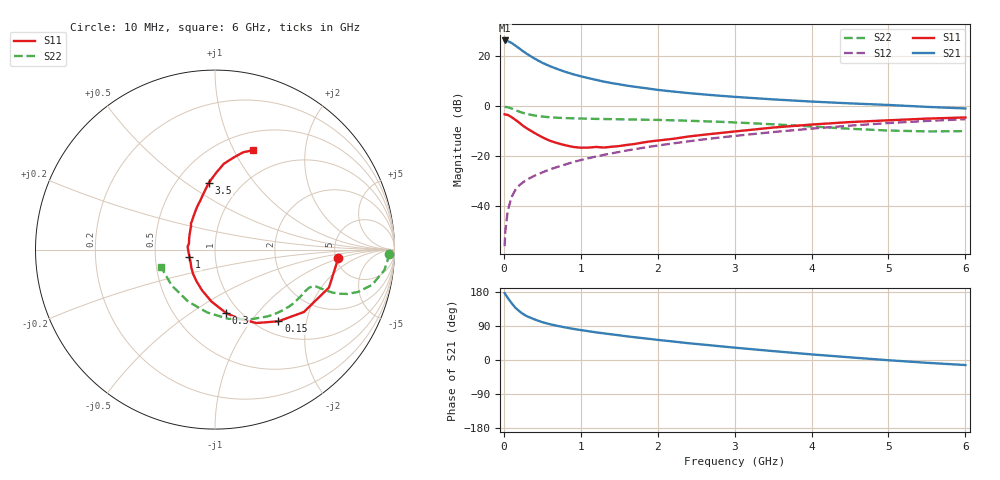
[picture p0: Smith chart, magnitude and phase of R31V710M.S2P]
! SIEMENS Small Signal Semiconductors
! BFR181
! Si NPN RF Bipolar Junction Transistor in SOT23
! VCE = 1.75 V  IC = 10 mA
! Common Emitter S-Parameters:  May  1996
# GHz  S  MA  R  50
!  f  S11  S21  S12  S22
! GHz  MAG  ANG  MAG  ANG  MAG  ANG  MAG  ANG
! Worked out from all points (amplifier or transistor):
!   36 points, 10 MHz to 6 GHz, reference 50 ohm
!   highest |S21| = 26.2 dB at 10 MHz (marker M1)
!   |S21| within 3 dB of that: start of sweep to 193.1 MHz
!   unconditionally stable (mu >= 1): 599.6 MHz to 2.801 GHz
!   at 250 MHz: K = 0.66, MSG = 26.2 dB, |S12| = -30.4 dB
!   at 1.4 GHz: K = 1.11, MAG = 12.0 dB, |S12| = -18.9 dB
!   at 6 GHz: K = 0.88, MSG = 2.1 dB, |S12| = -5.2 dB
!   S11 on the Smith chart (normalised r, x): 10 MHz: 5.23, -0.93; 150 MHz: 1.24, -1.38; 300 MHz: 0.87, -0.70; 1 GHz: 0.75, -0.06; 3.5 GHz: 0.71, +0.62; 6 GHz: 0.70, +1.20
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0.01  0.6877 -3.9  20.5 176.7  0.0016 92.2  0.9719 -1.3
0.02  0.6796 -7.6  20.31 173.3  0.0033 86.6  0.9658 -2.9
0.05  0.6693 -18.4  19.92 164.2  0.008 81.8  0.9508 -6.9
0.1  0.6049 -35.1  18.31 150.2  0.0153 76.0  0.8975 -12.6
0.15  0.5333 -48.5  16.16 137.9  0.0212 70.0  0.8334 -16.4
0.2  0.4692 -60.7  14.26 129.0  0.0262 67.9  0.7787 -18.5
0.25  0.4042 -71.3  12.48 121.3  0.0302 66.3  0.7331 -19.6
0.3  0.3592 -80.0  11.04 115.5  0.0341 66.2  0.6965 -20.1
0.4  0.2905 -93.8  8.902 107.1  0.0409 66.4  0.6499 -20.2
0.5  0.2389 -107.4  7.339 99.8  0.0475 67.2  0.6194 -20.1
0.6  0.2036 -120.7  6.27 94.5  0.0547 68.0  0.5992 -20.1
0.7  0.1816 -132.4  5.477 89.9  0.0614 68.8  0.586 -20.4
0.8  0.1654 -143.0  4.833 85.9  0.0684 68.9  0.5777 -20.8
1  0.1479 -164.4  3.945 79.0  0.0837 69.8  0.5651 -22.1
1.1  0.1485 -176.0  3.621 76.0  0.0913 70.2  0.5608 -23.1
1.3  0.149 166.5  3.089 70.3  0.1066 69.9  0.5533 -25.0
1.6  0.1683 146.3  2.567 62.4  0.1304 69.1  0.5436 -28.6
2.2  0.2226 122.2  1.958 48.8  0.1805 66.1  0.5212 -37.3
3.5  0.3737 95.3  1.364 23.5  0.304 55.3  0.4343 -63.9
4.5  0.4809 84.1  1.136 7.0  0.4084 43.6  0.3531 -97.0
5.5  0.5643 73.9  0.967 -7.4  0.5064 29.7  0.3133 -140.2
6  0.5942 68.9  0.9 -13.3  0.5486 22.2  0.3169 -162.6
